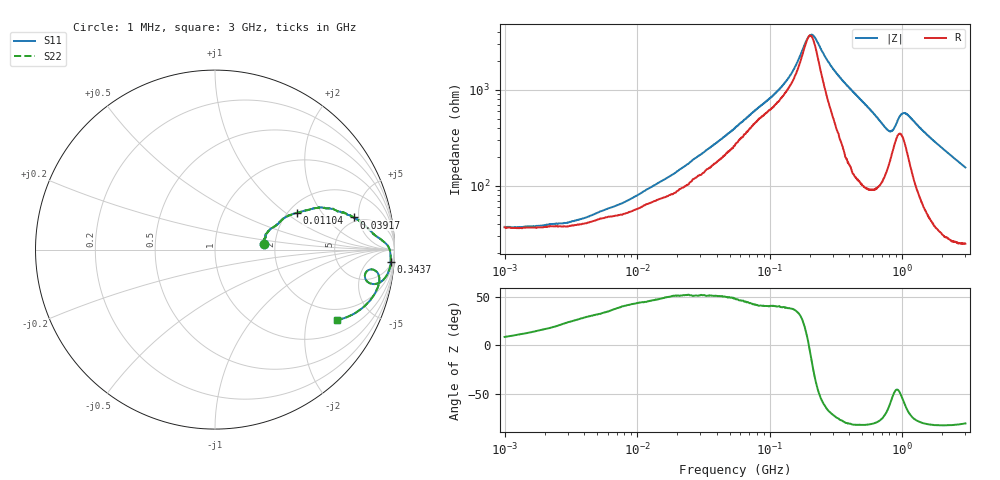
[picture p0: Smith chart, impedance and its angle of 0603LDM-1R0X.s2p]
!s-Parameter Generated by FASTRON Sdn. Bhd.
!FASTRON P/N : 0603LDM-1R0X
!Keysight Technologies: E4991B_MY54100416_A.01.15
!Date: Thu Nov 27 16:24:55 2025
!Version  :Rev00  Thu Nov 27 16:24:55 2025
!Data & Calibration Information:
!Freq  S11  S21  S12  S22
!PortZ  Port1:50+j0  Port2:50+j0
!When reading reference impedance value at option line is always used.
! Remarks : This data is being provided solely for informational purposes.
# Hz S dB R 50
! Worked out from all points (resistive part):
!   1601 points, 1 MHz to 3 GHz, reference 50 ohm
!   read as one part in series: R = 36.4 ohm at 1.041 MHz
!   S11 on the Smith chart (normalised r, x): 1 MHz: 1.74, +0.11; 11.04 MHz: 2.22, +1.21; 39.17 MHz: 4.45, +4.33; 343.7 MHz: 7, -26; 3 GHz: 1.49, -3.06
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1000000  -11.30 6.4  -2.72 -2.4  -2.72 -2.4  -11.30 6.4
3804036  -9.94 19.4  -3.00 -8.6  -3.00 -8.6  -9.94 19.4
1.104425e7  -6.02 24.2  -4.71 -20.7  -4.71 -20.7  -6.02 24.2
1.447069e7  -4.94 23.0  -5.55 -24.8  -5.55 -24.8  -4.94 23.0
2.362996e7  -3.24 19.2  -7.61 -32.9  -7.61 -32.9  -3.24 19.2
3.917023e7  -1.99 13.0  -10.80 -38.4  -10.80 -38.4  -1.99 13.0
5.504702e7  -1.43 9.0  -13.60 -39.2  -13.60 -39.2  -1.43 9.0
1.275944e8  -0.57 3.0  -21.80 -36.8  -21.80 -36.8  -0.57 3.0
1.527801e8  -0.41 2.0  -24.80 -35.2  -24.80 -35.2  -0.41 2.0
1.923242e8  -0.25 0.2  -30.90 -7.9  -30.90 -7.9  -0.25 0.2
2.083556e8  -0.22 -0.4  -31.70 16.9  -31.70 16.9  -0.22 -0.4
2.234756e8  -0.20 -1.0  -30.80 37.5  -30.80 37.5  -0.20 -1.0
2.799137e8  -0.18 -2.7  -25.90 65.4  -25.90 65.4  -0.18 -2.7
3.436571e8  -0.17 -4.2  -22.60 73.1  -22.60 73.1  -0.17 -4.2
5.929311e8  -0.34 -9.2  -15.80 71.9  -15.80 71.9  -0.34 -9.2
7.925923e8  -1.16 -12.1  -12.60 51.8  -12.60 51.8  -1.16 -12.1
8.458658e8  -1.42 -10.3  -13.00 42.8  -13.00 42.8  -1.42 -10.3
9.209708e8  -1.27 -7.5  -14.80 38.2  -14.80 38.2  -1.27 -7.5
9.828732e8  -0.99 -7.3  -15.90 44.7  -15.90 44.7  -0.99 -7.3
1.048936e9  -0.78 -8.1  -15.90 53.4  -15.90 53.4  -0.78 -8.1
1.67054e9  -0.77 -17.1  -10.50 65.0  -10.50 65.0  -0.77 -17.1
3e9  -2.10 -30.0  -5.91 50.8  -5.91 50.8  -2.10 -30.0
